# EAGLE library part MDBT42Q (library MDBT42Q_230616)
Raytac Corporation Part Number: (nRF52832) MDBT42Q-512KV2 / MDBT42Q-P512KV2 / MDBT42Q-U512KV2 (nRF52810) MDBT42Q-192KV2 / MDBT42Q-P192KV2 (nRF52811) MDBT42Q-192KL / MDBT42Q-P192KL Bluetooth Low Energy Module based on Noridc nRF52832 / nRF52810 / nRF52811 Size: 16x10mm Source: Raytac datasheet
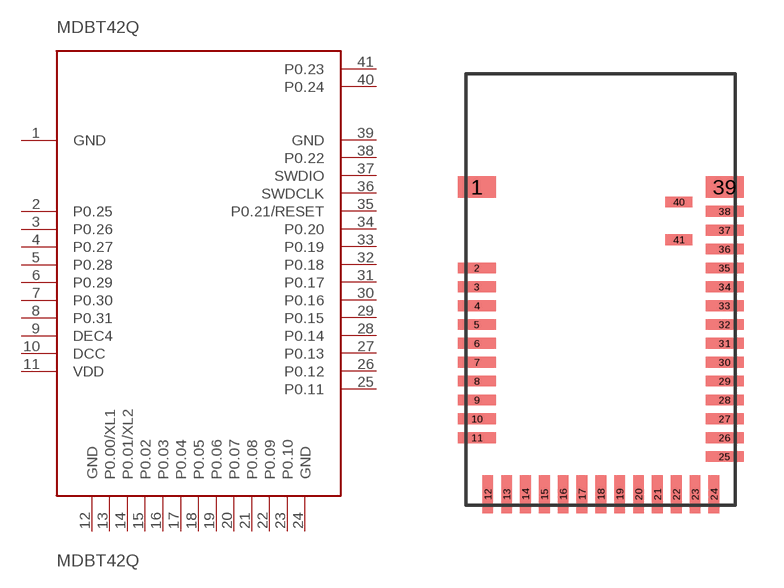
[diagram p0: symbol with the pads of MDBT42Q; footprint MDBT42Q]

Designator prefix MDBT42Q

## MDBT42Q  [MDBT42Q]
1  GND
2  P0.25
3  P0.26
4  P0.27
5  P0.28
6  P0.29
7  P0.30
8  P0.31
9  DEC4
10  DCC
11  VDD
12  GND
13  P0.00/XL1
14  P0.01/XL2
15  P0.02
16  P0.03
17  P0.04
18  P0.05
19  P0.06
20  P0.07
21  P0.08
22  P0.09
23  P0.10
24  GND
25  P0.11
26  P0.12
27  P0.13
28  P0.14
29  P0.15
30  P0.16
31  P0.17
32  P0.18
33  P0.19
34  P0.20
35  P0.21/RESET
36  SWDCLK
37  SWDIO
38  P0.22
39  GND
40  P0.24
41  P0.23

## Footprint MDBT42Q (pad centres in mm)
Raytac Corporation Part Number: (nRF52832) MDBT42Q-512KV2 / MDBT42Q-P512KV2 (nRF52810) MDBT42Q-192KV2 / MDBT42Q-P192KV2 (nRF52811) MDBT42Q-192KL / MDBT42Q-P192KL Bluetooth Low Energy Module based on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
smd 1.4 x 0.8: 1 -4.6,3.8; 39 4.6,3.8
smd 1.4 x 0.4: 2 -4.6,0.8; 3 -4.6,0.1; 4 -4.6,-0.6; 5 -4.6,-1.3; 6 -4.6,-2; 7 -4.6,-2.7; 8 -4.6,-3.4; 9 -4.6,-4.1; 10 -4.6,-4.8; 11 -4.6,-5.5; 25 4.6,-6.2; 26 4.6,-5.5; 27 4.6,-4.8; 28 4.6,-4.1; 29 4.6,-3.4; 30 4.6,-2.7; 31 4.6,-2; 32 4.6,-1.3; 33 4.6,-0.6; 34 4.6,0.1; 35 4.6,0.8; 36 4.6,1.5; 37 4.6,2.2; 38 4.6,2.9
smd 0.4 x 1.4: 12 -4.2,-7.6; 13 -3.5,-7.6; 14 -2.8,-7.6; 15 -2.1,-7.6; 16 -1.4,-7.6; 17 -0.7,-7.6; 18 0,-7.6; 19 0.7,-7.6; 20 1.4,-7.6; 21 2.1,-7.6; 22 2.8,-7.6; 23 3.5,-7.6; 24 4.2,-7.6
smd 1 x 0.4: 40 2.9,3.25; 41 2.9,1.85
